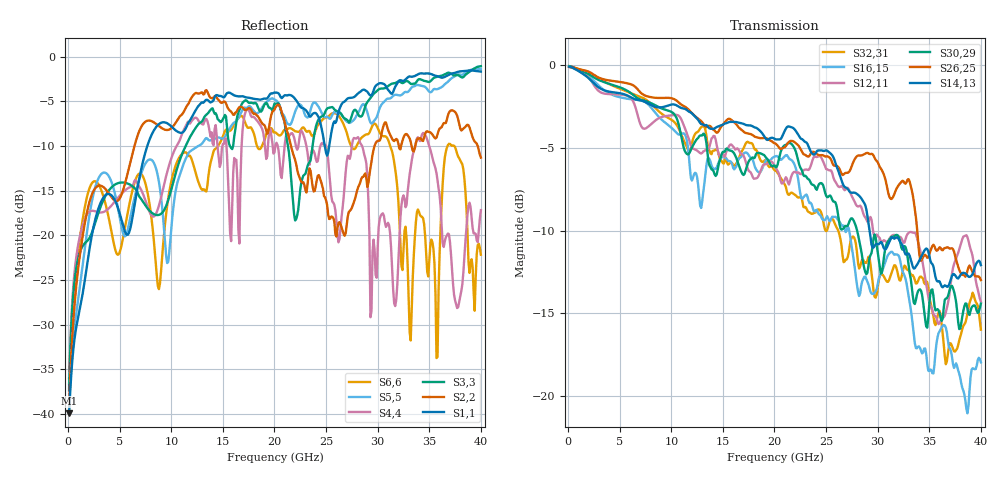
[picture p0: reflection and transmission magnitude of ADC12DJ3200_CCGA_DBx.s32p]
! Touchstone file
! Texas Instruments 4/21/2021
! ADC12DJ3200QML-SP
! Package-type  CCGA [BGA]
! pins/pkg drawing  196-pin NWE
! CCGA Ceramic Package with columns (ceramic column grid array)
! High-speed serialized data output for channel B, lane 0-7
# GHZ S MA R 50.000000
! Port[1] = DB0N_BGA_J14
! Port[2] = DB0N_DIE_6
! Port[3] = DB0P_BGA_K14
! Port[4] = DB0P_DIE_5
! Port[5] = DB1N_BGA_L14
! Port[6] = DB1N_DIE_8
! Port[7] = DB1P_BGA_M14
! Port[8] = DB1P_DIE_7
! Port[9] = DB2N_BGA_P13
! Port[10] = DB2N_DIE_10
! Port[11] = DB2P_BGA_P12
! Port[12] = DB2P_DIE_9
! Port[13] = DB3N_BGA_P11
! Port[14] = DB3N_DIE_12
! Port[15] = DB3P_BGA_P10
! Port[16] = DB3P_DIE_11
! Port[17] = DB4N_BGA_J13
! Port[18] = DB4N_DIE_14
! Port[19] = DB4P_BGA_K13
! Port[20] = DB4P_DIE_13
! Port[21] = DB5N_BGA_L13
! Port[22] = DB5N_DIE_16
! Port[23] = DB5P_BGA_M13
! Port[24] = DB5P_DIE_15
! Port[25] = DB6N_BGA_N13
! Port[26] = DB6N_DIE_18
! Port[27] = DB6P_BGA_N12
! Port[28] = DB6P_DIE_17
! Port[29] = DB7N_BGA_N11
! Port[30] = DB7N_DIE_20
! Port[31] = DB7P_BGA_N10
! Port[32] = DB7P_DIE_19
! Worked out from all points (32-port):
!   400 points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, 100 MHz to 40 GHz, reference 50 ohm
!   strongest paths, dB at 100 MHz, 10.1 GHz, 20.1 GHz, 30.1 GHz, 40 GHz:
!     S14,13: -0.1, -2.4, -4.5, -10.8, -12.1
!     S26,25: -0.1, -2.0, -4.7, -6.0, -13.0
!     S30,29: -0.1, -2.9, -6.2, -11.8, -14.4
!     S12,11: -0.1, -3.0, -6.2, -10.4, -14.3
!     S16,15: -0.1, -3.8, -5.5, -12.9, -18.0
!     S32,31: -0.1, -3.3, -6.4, -13.0, -16.0
!   lowest |S11| = -39.9 dB at 100 MHz (marker M1), VSWR 1.02, Z = 50.9 + j0.502 ohm
!   |S11| at or under -10 dB: start of sweep to 7.676 GHz; 24.87 GHz to 25.3 GHz (430.1 MHz wide, 1.71 % of centre)
